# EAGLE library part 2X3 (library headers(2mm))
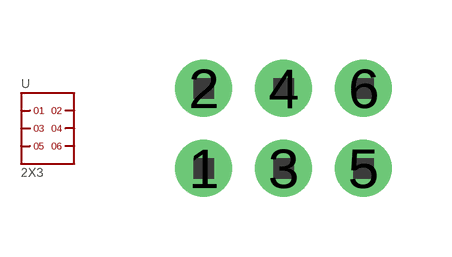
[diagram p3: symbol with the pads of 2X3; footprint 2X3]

Designator prefix -

## 2X3  [2X3]
1  1
2  2
3  3
4  4
5  5
6  6

## Footprint 2X3 (pad centres in mm)
drill 0.8 pad 1.422: 1 -2,-1; 2 -2,1; 3 0,-1; 4 0,1; 5 2,-1; 6 2,1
